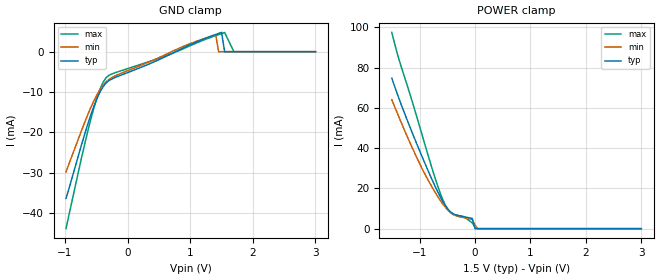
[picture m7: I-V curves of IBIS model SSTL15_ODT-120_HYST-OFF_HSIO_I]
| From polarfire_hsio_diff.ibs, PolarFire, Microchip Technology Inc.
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|   Model SSTL15_ODT-120_HYST-OFF_HSIO_I
[Model]   SSTL15_ODT-120_HYST-OFF_HSIO_I
Model_type   Input
Vinl =   0.65
Vinh =   0.85
|   typ   min   max
C_comp_pullup   1.335e-12   1.335e-12   1.380e-12
C_comp_pulldown  1.335e-12   1.335e-12   1.380e-12
[Temperature Range]  25C   100C   -40C
[Voltage Range]  1.5   1.425   1.575
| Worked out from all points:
|   POWER clamp passes 1 mA (typ) near -0.01 V on its own axis
[GND Clamp]
| Voltage   I(typ)   I(min)   I(max)
-984.4mV  -36.37mA   -29.8mA    -43.85mA
-738.3mV  -23.16mA   -19.61mA   -26.39mA
-541.4mV  -13.61mA   -12.24mA   -14.07mA
-393.7mV  -8.729mA   -8.343mA   -7.615mA
-295.3mV  -7.121mA   -6.832mA   -5.812mA
937.5mV   1.297mA    1.625mA    1.065mA
1.406V    4.248mA    4.224mA    3.981mA
1.453V    4.515mA    0A         4.235mA
1.5V      4.781mA    0A         4.487mA
1.549V    0A         0A         4.753mA
1.697V    0A         0A         0A
3V        0A         0A         0A
[POWER Clamp]
| Voltage   I(typ)   I(min)   I(max)
-1.5V     74.73mA    64.02mA    97.44mA
-1.378V   65.14mA    55.84mA    84.7mA
-1.034V   41mA       34.32mA    54.06mA
-885.9mV  31.34mA    26.2mA     40.18mA
-689.1mV  19.28mA    16.73mA    22.55mA
-541.4mV  11.74mA    10.87mA    12.02mA
-443mV    8.344mA    8.011mA    8.082mA
-196.9mV  5.897mA    5.399mA    5.946mA
-49.22mV  5.061mA    4.59mA     2.817mA
0V        0A         1.79mA     968.3uA
46.88mV   0A         0A         0A
3V        0A         0A         0A
